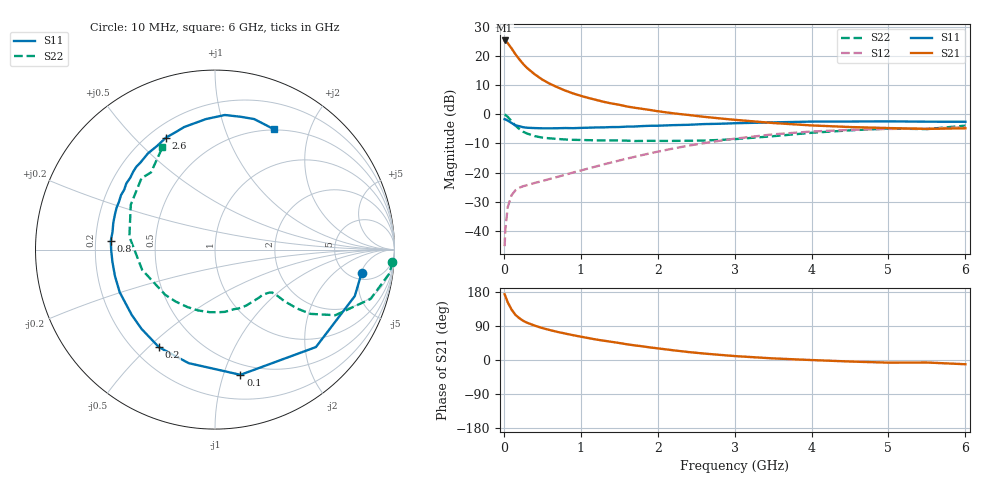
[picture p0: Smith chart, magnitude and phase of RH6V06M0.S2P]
! SIEMENS Small Signal Semiconductors
! BFR106
! Si NPN RF Bipolar Junction Transistor in SOT23
! VCE = 6 V  IC = 6 mA
! Common Emitter S-Parameters:  August  1996
# GHz  S  MA  R  50
!  f  S11  S21  S12  S22
! GHz  MAG  ANG  MAG  ANG  MAG  ANG  MAG  ANG
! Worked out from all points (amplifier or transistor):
!   36 points, 10 MHz to 6 GHz, reference 50 ohm
!   highest |S21| = 25.4 dB at 10 MHz (marker M1)
!   |S21| within 3 dB of that: start of sweep to 107.1 MHz
!   unconditionally stable (mu >= 1): 583.5 MHz to 1.862 GHz; 5.05 GHz to end of sweep
!   at 250 MHz: K = 0.56, MSG = 21.1 dB, |S12| = -24.7 dB
!   at 1.4 GHz: K = 1.12, MAG = 8.1 dB, |S12| = -16.5 dB
!   at 6 GHz: K = 1.02, MAG = -1.0 dB, |S12| = -4.4 dB
!   S11 on the Smith chart (normalised r, x): 10 MHz: 6.17, -5.16; 100 MHz: 0.40, -1.14; 200 MHz: 0.30, -0.54; 800 MHz: 0.26, +0.04; 2.6 GHz: 0.27, +0.62; 6 GHz: 0.49, +1.49
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0.01  0.8269 -9.2  18.72 173.5  0.0054 84.6  0.991 -3.9
0.02  0.8208 -18.4  18.51 168.4  0.0106 79.4  0.9816 -7.7
0.05  0.7817 -44.0  16.85 152.4  0.0252 68.8  0.9095 -17.6
0.1  0.7119 -78.5  13.7 133.3  0.0406 55.1  0.7636 -28.6
0.15  0.6494 -103.1  10.88 119.3  0.0494 46.5  0.642 -33.9
0.2  0.627 -119.9  8.92 110.6  0.0546 43.5  0.5618 -35.7
0.25  0.6021 -132.9  7.4 103.5  0.058 41.6  0.5044 -36.3
0.3  0.5896 -141.9  6.325 98.6  0.0605 42.2  0.4693 -36.6
0.4  0.5817 -155.9  4.91 90.8  0.0661 43.5  0.423 -36.5
0.5  0.5765 -165.2  3.971 84.3  0.0714 46.4  0.3987 -36.9
0.6  0.5756 -173.1  3.354 78.9  0.0776 48.8  0.3867 -38.2
0.8  0.5826 175.2  2.567 69.7  0.0917 54.1  0.3699 -42.2
1.1  0.5904 161.1  1.917 57.8  0.1176 60.2  0.3602 -50.6
1.3  0.598 153.2  1.643 50.9  0.1382 62.5  0.3567 -57.0
1.6  0.6166 143.2  1.368 41.5  0.1735 63.8  0.3531 -68.3
2.2  0.6533 124.9  1.045 25.7  0.2585 60.7  0.3499 -94.7
2.6  0.6813 113.6  0.909 17.1  0.3197 55.6  0.355 -115.6
3.5  0.7289 94.0  0.711 4.2  0.4535 39.8  0.4214 -164.5
4.5  0.7538 79.0  0.606 -4.0  0.5409 20.3  0.5318 151.9
5  0.7593 73.3  0.582 -7.0  0.562 12.0  0.571 135.8
5.5  0.7492 67.4  0.563 -6.6  0.5701 7.7  0.5587 129.7
6  0.7462 63.9  0.577 -11.2  0.6014 -0.4  0.6405 117.2
